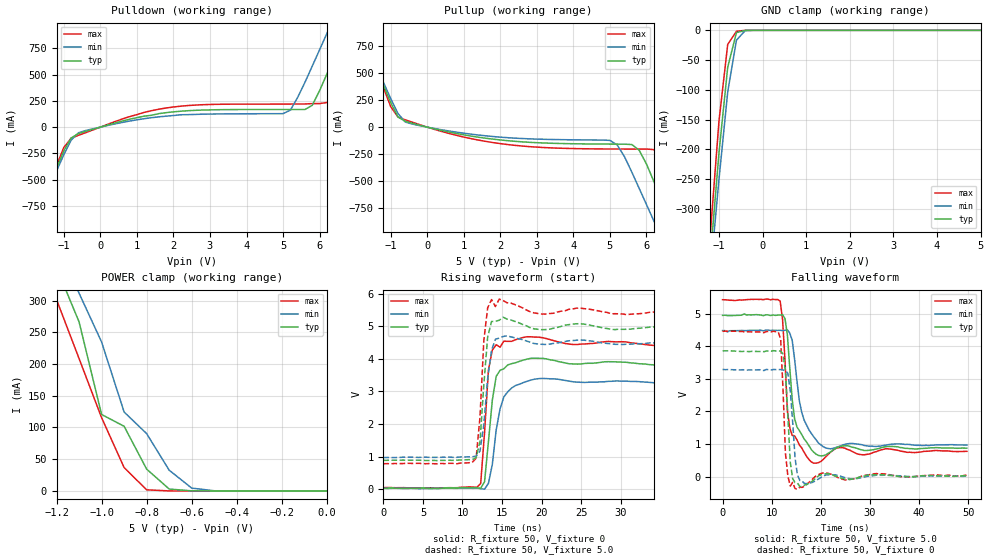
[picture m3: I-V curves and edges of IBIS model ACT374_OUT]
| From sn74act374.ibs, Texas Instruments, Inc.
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|   Model ACT374_OUT
[Model]   ACT374_OUT
Model_type  3-state
Polarity   Non-Inverting
Enable   Active-Low
Vmeas = 1.5v
Cref = 50pf
Rref = 500
Vref = 0V
| variable   typ   min   max
C_comp   8.0pF   NA   NA
[Temperature Range]   40   100   -40
| Ambient temperature   25   85   -40
[Voltage range]   5.0   4.5   5.5
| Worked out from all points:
|   slope of the pulldown table from 0 to 0.75 V, typ, clamps not added: 10.6 ohm
|   slope of the pullup table from 0 to 0.75 V, typ, clamps not added: 13.5 ohm
|   GND clamp passes 1 mA (typ) near -0.45 V on its own axis
|   POWER clamp passes 1 mA (typ) near -0.63 V on its own axis
|   rising waveform, R_fixture 50, V_fixture 0: 20-80 % time 992ps typ, 1.26ns min, 723ps max; typ from 0.025 V to 3.85 V
|   falling waveform, R_fixture 50, V_fixture 5.0: 20-80 % time 1.54ns typ, 2.3ns min, 1.14ns max; typ from 4.95 V to 0.871 V
|   rising waveform, R_fixture 50, V_fixture 5.0: 20-80 % time 725ps typ, 882ps min, 668ps max; typ from 0.882 V to 4.94 V
|   falling waveform, R_fixture 50, V_fixture 0: 20-80 % time 805ps typ, 931ps min, 722ps max; typ from 3.86 V to 0.026 V
[Pulldown]
|   Voltage   I(typ)   I(min)   I(max)
-5V       -3.797A    -3.423A    -4.218A
-1.8V     -932mA     -893.5mA   -971.2mA
-1V       -225mA     -261.7mA   -193.4mA
-600mV    -61.29mA   -53.45mA   -78.04mA
1.8V      137.8mA    104.7mA    182.1mA
5.2V      167.8mA    161.6mA    219.7mA
5.8V      208.2mA    580.9mA    224mA
6.2V      505.1mA    891mA      234mA
6.4V      670.6mA    1.046A     266.6mA
6.8V      1.001A     1.356A     596mA
7.2V      1.332A     1.666A     939.3mA
10V       3.648A     3.837A     3.343A
[Pullup]
|   Voltage   I(typ)   I(min)   I(max)
-5V       3.637A     3.358A     3.97A
-1.8V     903.6mA    881.7mA    931.6mA
-1V       227.8mA    265.3mA    190.4mA
-600mV    53.95mA    47.07mA    67.8mA
2V        -119mA     -92.86mA   -152.9mA
5V        -157.5mA   -123.1mA   -202.9mA
5.4V      -158mA     -275mA     -203.4mA
5.8V      -213.9mA   -567.6mA   -203.4mA
6.4V      -668.7mA   -1.019A    -276.4mA
6.8V      -1.002A    -1.32A     -609.3mA
7.2V      -1.335A    -1.62A     -977.2mA
10V       -3.668A    -3.726A    -3.553A
[GND Clamp]
|   Voltage   I(typ)   I(min)   I(max)
-5V       -3.833A    -3.438A    -4.283A
-1.2V     -382.4mA   -409.7mA   -342.9mA
-1V       -205.5mA   -250.2mA   -152.1mA
-800mV    -61.96mA   -103.5mA   -23.66mA
-600mV    -3.843mA   -16.55mA   -1.603mA
-400mV    -146uA     -527.2uA   -20.41uA
5V        117.1pA    4.541nA    -259.8pA
[POWER Clamp]
|   Voltage   I(typ)   I(min)   I(max)
-5V       3.844A     3.501A     4.213A
-1.3V     440.4mA    473.7mA    398mA
-1.2V     352mA      391.8mA    301.6mA
-1.1V     266.6mA    311.7mA    208.7mA
-1V       120.5mA    234.8mA    115.5mA
-900mV    101.9mA    124.4mA    36.82mA
-800mV    34.39mA    90.32mA    1.714mA
-700mV    2.98mA     32.7mA     24.63uA
-600mV    95.58uA    4.463mA    215.6nA
-500mV    2.289uA    264.9uA    2.739nA
0V        -199.1pA   3.26nA     82.88pA
[Ramp]
| variable   typ   min   max
dV/dt_r  2.334E+00/9.200E-10  1.965E+00/1.190E-09  2.712E+00/6.330E-10
dV/dt_f  2.518E+00/1.522E-09  2.088E+00/2.286E-09  2.790E+00/1.038E-09
R_load = 50
[Rising Waveform]
R_fixture = 50
V_fixture = 0
V_fixture_min = 0
V_fixture_max = 0
C_fixture = 0pf
L_fixture = 0nH
|   Time   V(typ)   V(min)   V(max)
0s        24.74mV    24.28mV    45.95mV
12.3ns    25.96mV    12.08mV    172.8mV
12.79ns   226.8mV    -2.724mV   1.746V
13.28ns   1.46V      176.3mV    3.66V
13.77ns   2.73V      757.3mV    4.275V
14.26ns   3.464V     1.819V     4.436V
15.23ns   3.699V     2.834V     4.546V
20.12ns   4.019V     3.402V     4.652V
24.02ns   3.848V     3.297V     4.443V
50ns      3.848V     3.276V     4.458V
[Falling Waveform]
R_fixture = 50
V_fixture = 5.0
V_fixture_min = 4.5
V_fixture_max = 5.5
C_fixture = 0pf
L_fixture = 0nH
|   Time   V(typ)   V(min)   V(max)
0s        4.946V     4.478V     5.426V
11.72ns   4.957V     4.488V     5.382V
12.7ns    4.847V     4.488V     3.572V
13.18ns   4.358V     4.503V     2.023V
13.67ns   3.336V     4.4V       1.499V
14.65ns   1.778V     3.605V     1.251V
16.11ns   1.288V     1.966V     876.6mV
18.07ns   824.8mV    1.323V     447.8mV
21.97ns   757.1mV    850.8mV    747.8mV
49.71ns   870.9mV    965.8mV    773.9mV
[Rising Waveform]
R_fixture = 50
V_fixture = 5.0
V_fixture_min = 4.5
V_fixture_max = 5.5
C_fixture = 0pf
L_fixture = 0nH
|   Time   V(typ)   V(min)   V(max)
0s        882.4mV    968.6mV    778.9mV
11.72ns   963.8mV    1.014V     946mV
12.21ns   1.455V     1.166V     2.212V
12.7ns    3.213V     1.988V     4.572V
13.18ns   4.672V     3.391V     5.57V
13.67ns   5.15V      4.262V     5.826V
14.16ns   5.159V     4.605V     5.611V
15.63ns   5.225V     4.711V     5.727V
20.02ns   4.901V     4.45V      5.381V
49.71ns   4.941V     4.466V     5.41V
[Falling Waveform]
R_fixture = 50
V_fixture = 0
V_fixture_min = 0
V_fixture_max = 0
C_fixture = 0pf
L_fixture = 0nH
|   Time   V(typ)   V(min)   V(max)
0s        3.859V     3.287V     4.457V
11.33ns   3.855V     3.282V     4.439V
11.82ns   3.849V     3.282V     4.214V
12.79ns   3.251V     3.254V     721.5mV
13.77ns   446.2mV    2.641V     -293mV
14.75ns   -186mV     566.9mV    -369.1mV
15.23ns   -200.5mV   50.99mV    -386.9mV
16.7ns    -258.3mV   -214.1mV   -288.2mV
20.61ns   75.86mV    18.64mV    115.4mV
50ns      25.96mV    12.99mV    30.24mV
